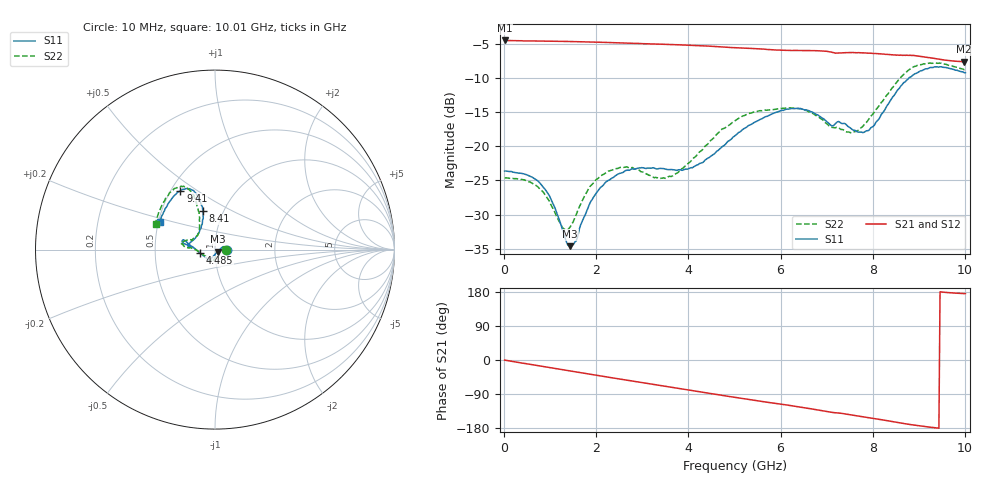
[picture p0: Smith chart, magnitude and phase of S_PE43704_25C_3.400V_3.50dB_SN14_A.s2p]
! Device ID: PE43704
! Dir: z:\PE43704\PE43704_Char_1_20130516\PE43704\AMB\3p400V\3p50dB
! Serial: 14
! Insertion: A
! Impedance: 50 ohm
! Temp: Amb
! VDD: 3.400V
! Attenuation Step: 3.50dB
! IDD: 1.140560e-01mA
#  Hz  S  RI  R  50
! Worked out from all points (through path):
!   401 points, 10 MHz to 10.01 GHz, reference 50 ohm
!   highest |S21| = -4.52 dB at 10 MHz (marker M1); lowest = -7.6 dB at 9.985 GHz (marker M2)
!   group delay of S21, straight-line fit = 52.6 ps
!   lowest |S11| = -34.6 dB at 1.435 GHz (marker M3), VSWR 1.04, Z = 51.4 - j1.25 ohm
!   |S11| at or under -10 dB: start of sweep to 8.783 GHz
!   |S22| runs from -32.2 to -7.8 dB; largest |S21 - S12| = 0.0045
!   S11 on the Smith chart (normalised r, x): 10 MHz: 1.14, +0.00; 4.485 GHz: 0.85, -0.04; 8.41 GHz: 0.80, +0.36; 9.41 GHz: 0.56, +0.43; 10.01 GHz: 0.51, +0.18
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1e7  0.0658 0.000174  0.5941 -0.00237  0.5943 -0.00228  0.0586 0.000285
7.85e8  0.0501 0.0184  0.5656 -0.1612  0.5656 -0.1609  0.046 0.0146
1.26e9  0.025 -0.000675  0.5285 -0.2516  0.5286 -0.2514  0.0243 -0.00774
1.435e9  0.014 -0.0122  0.5109 -0.2824  0.5107 -0.2823  0.0156 -0.0205
1.685e9  -0.000363 -0.0277  0.4822 -0.3249  0.4823 -0.3247  0.00421 -0.039
1.935e9  -0.012 -0.0405  0.4498 -0.3635  0.45 -0.3634  -0.00456 -0.0536
2.26e9  -0.0227 -0.0515  0.4032 -0.4086  0.4033 -0.4083  -0.0134 -0.0644
2.735e9  -0.0323 -0.059  0.3279 -0.4626  0.3281 -0.4626  -0.0235 -0.0653
3.36e9  -0.0368 -0.0581  0.2201 -0.5128  0.2207 -0.5126  -0.0294 -0.0503
3.735e9  -0.0456 -0.0487  0.1518 -0.5317  0.1525 -0.5315  -0.0507 -0.0377
4.485e9  -0.0821 -0.0206  0.0117 -0.5388  0.0123 -0.5394  -0.1105 0.000472
5.01e9  -0.1189 0.0103  -0.0782 -0.52  -0.0781 -0.5202  -0.1535 0.0105
5.985e9  -0.1735 0.0532  -0.2228 -0.4532  -0.2205 -0.4535  -0.1861 0.0327
6.685e9  -0.1748 0.0347  -0.3175 -0.3871  -0.3177 -0.3864  -0.1672 0.0491
7.585e9  -0.119 0.0548  -0.4013 -0.2715  -0.401 -0.2712  -0.0934 0.086
7.96e9  -0.0857 0.1065  -0.4272 -0.2158  -0.4274 -0.2175  -0.0861 0.1421
8.36e9  -0.0662 0.1987  -0.4427 -0.1515  -0.4421 -0.1536  -0.0945 0.2309
8.41e9  -0.0674 0.2129  -0.4443 -0.1432  -0.4439 -0.1449  -0.1003 0.2445
8.86e9  -0.1054 0.3118  -0.4559 -0.0713  -0.4528 -0.0728  -0.1543 0.3433
9.41e9  -0.1923 0.3267  -0.4351 -0.00275  -0.4349 -0.00179  -0.2375 0.3275
9.985e9  -0.3022 0.1671  -0.4137 0.0346  -0.415 0.0362  -0.3278 0.1539
1.001e10  -0.3071 0.1559  -0.4152 0.0353  -0.417 0.0356  -0.3308 0.145
